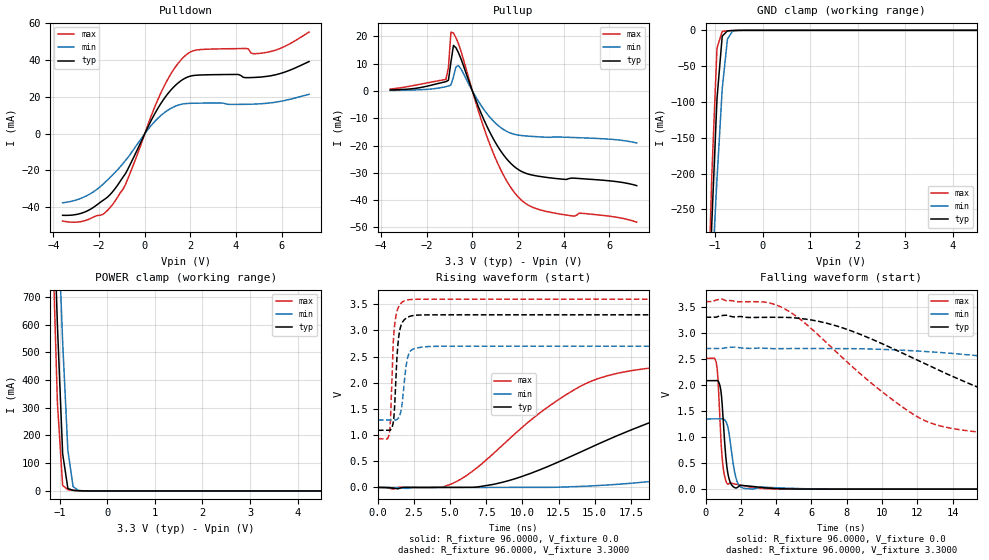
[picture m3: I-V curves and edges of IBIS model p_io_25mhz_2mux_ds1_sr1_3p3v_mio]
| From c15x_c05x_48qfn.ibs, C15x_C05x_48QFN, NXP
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[Model] p_io_25mhz_2mux_ds1_sr1_3p3v_mio
|   Model p_io_25mhz_2mux_ds1_sr1_3p3v_mio
| This model was characterised for following simulation conditions:
| External (pad) voltage:
|   - Typ: 3.3V,   - Min: 2.7V,   - Max: 3.6V
| Library cells for typ/min/max conditions are connected as defined below:
|  pad - External Pad
|  ipp_do_lv - Core Input
|  ipp_obe_lv - Output Buffer Enable
|  IOGC - NC
|  REFH3V3 - REFH3V3
|  REFL3V3 - REFL3V3
|  ZI - NC
|  abut_ncal_vddio[1] - vddio
|  abut_ncal_vddio[2] - vddio
|  abut_ncal_vddio[3] - vssio
|  abut_ncal_vddio[4] - vddio
|  abut_ncal_vddio[5] - vddio
|  abut_ncal_vddio[6] - vssio
|  abut_pcal_vddio[1] - vssio
|  abut_pcal_vddio[2] - vssio
|  abut_pcal_vddio[3] - vddio
|  abut_pcal_vddio[4] - vssio
|  abut_pcal_vddio[5] - vssio
|  abut_pcal_vddio[6] - vddio
|  ipp_do_1p8v - ipp_do_1p8v
|  ipp_dse_lv - vdd_lv
|  ipp_eftd_lv - NC
|  ipp_ina_mux_vddio - NC
|  ipp_ina_mux_vddio[0] - NC
|  ipp_ina_mux_vddio[1] - NC
|  ipp_ina_r0_vddio - NC
|  ipp_ina_r0a_vddio - NC
|  ipp_ina_r0b_vddio - NC
|  ipp_ina_r0c_vddio - NC
|  ipp_ina_r0d_vddio - NC
|  ipp_ina_r0e_vddio - NC
|  ipp_ina_r0f_vddio - NC
|  ipp_ina_r300_vddio - NC
|  ipp_ina_r300a_vddio - NC
|  ipp_ina_r300b_vddio - NC
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Model_type I/O
Polarity   Non-Inverting
Enable   Active-High
Vinl =   0.9900V
Vinh =   2.3100V
Vmeas =  1.6500V
Cref =   30.0000pF
Rref =   1.0000M
Vref =   3.3000V
C_comp   1.2811pF   1.2303pF   1.3501pF
|C_comp_pullup   0.5368pF   0.5680pF   0.5155pF
|C_comp_pulldown   0.6706pF   0.7073pF   0.6415pF
[Model Spec]
| variable   typ   min   max
Vinh   2.3100V   1.8900V   2.5200V
Vinl   0.9900V   0.8100V   1.0800V
[Temperature Range]   25.0000   0.1250k   -40.0000
[Voltage Range]   3.3000V   2.7000V   3.6000V
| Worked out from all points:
|   slope of the pulldown table from 0 to 0.495 V, typ, clamps not added: 40.8 ohm
|   slope of the pullup table from 0 to 0.495 V, typ, clamps not added: 47.8 ohm
|   GND clamp passes 1 mA (typ) near -0.74 V on its own axis
|   POWER clamp passes 1 mA (typ) near -0.62 V on its own axis
|   rising waveform, R_fixture 96.0000, V_fixture 0.0: 20-80 % time 12ns typ, 25.5ns min, 7.17ns max; typ from 0 V to 2.08 V
|   rising waveform, R_fixture 96.0000, V_fixture 3.3000: 20-80 % time 277ps typ, 348ps min, 248ps max; typ from 1.09 V to 3.3 V
|   falling waveform, R_fixture 96.0000, V_fixture 0.0: 20-80 % time 280ps typ, 355ps min, 248ps max; typ from 2.08 V to 0 V
|   falling waveform, R_fixture 96.0000, V_fixture 3.3000: 20-80 % time 9.25ns typ, 20.1ns min, 5.6ns max; typ from 3.3 V to 1.09 V
[Pulldown]
|Voltage   I(typ)   I(min)   I(max)
-3.6V     -44.37mA   -37.58mA   -47.51mA
-2.5V     -41.88mA   -33.45mA   -46.76mA
-1.84V    -36.35mA   -27.58mA   -43.92mA
-1.4V     -31.43mA   -22.29mA   -38.34mA
-850mV    -21.79mA   -14.63mA   -27.74mA
800mV     18.21mA    10.89mA    24.66mA
1.35V     26.41mA    15.03mA    36.45mA
1.9V      30.96mA    16.49mA    43.73mA
4.43V     30.52mA    16mA       46.39mA
4.76V     30.6mA     16.11mA    43.53mA
5.31V     31.15mA    16.53mA    44.19mA
7.2V      39.28mA    21.46mA    55.3mA
[Pullup]
|Voltage   I(typ)   I(min)   I(max)
-3.6V     375uA      207.1uA    721uA
-1.16V    3.419mA    1.608mA    4.218mA
-1.05V    3.929mA    1.825mA    8.684mA
-940mV    10.66mA    2.209mA    21.58mA
-830mV    16.7mA     5.227mA    21.23mA
-720mV    15.82mA    8.86mA     19.48mA
-610mV    14mA       9.299mA    17.3mA
820mV     -16.02mA   -10.13mA   -20.76mA
1.48V     -24.66mA   -14.68mA   -32.62mA
2.03V     -28.88mA   -16.19mA   -39.03mA
3.35V     -31.76mA   -16.97mA   -44.31mA
7.2V      -34.67mA   -19.04mA   -48.06mA
[GND_clamp]
|Voltage   I(typ)   I(min)   I(max)
-3.6V     -5.309A    -4.128A    -6.876A
-1.18V    -466mA     -495.4mA   -458.9mA
-1.07V    -271.1mA   -348.5mA   -204.6mA
-960mV    -95.65mA   -208mA     -24.74mA
-850mV    -8.096mA   -81.85mA   -1.471mA
-740mV    -719.7uA   -12.14mA   -717.6uA
-630mV    -272.5uA   -923.5uA   -300.8uA
-300mV    -385.6nA   -2.502uA   -74.88nA
7.2V      0A         0A         0A
[POWER_clamp]
|Voltage   I(typ)   I(min)   I(max)
-3.6V     14.48A     12.95A     16.35A
-1.16V    1.177A     1.535A     951.2mA
-1.05V    598.4mA    1.032A     318mA
-940mV    134.2mA    537.3mA    20.02mA
-830mV    8.708mA    145.4mA    4.242mA
-720mV    2.127mA    15.38mA    2.218mA
-610mV    847.4uA    1.853mA    834.1uA
7.2V      0A         0A         0A
[Ramp]
| variable   typ   min   max
dV/dt_r  1.2491/12.0373n   0.8026/25.5375n   1.5061/7.1717n
dV/dt_f  1.3249/9.2469n   0.8437/20.0855n   1.6024/5.6005n
R_load = 96.0000
[Rising Waveform]
R_fixture= 96.0000
V_fixture= 0.0
V_fixture_min= 0.0
V_fixture_max= 0.0
|time   V(typ)   V(min)   V(max)
0s        3.081nV    103.2nV    10.53nV
4.572ns   -81.02uV   -467uV     15.01mV
8.528ns   91.84mV    7.678uV    783.2mV
11.66ns   388.3mV    693.5uV    1.518V
14.79ns   773.2mV    29.16mV    2.034V
21.68ns   1.514V     196.4mV    2.356V
30.99ns   1.882V     534.2mV    2.456V
42.83ns   2.003V     937.6mV    2.493V
53.59ns   2.045V     1.127V     2.504V
127.4ns   2.082V     1.338V     2.51V
[Rising Waveform]
R_fixture= 96.0000
V_fixture= 3.3000
V_fixture_min= 2.7000
V_fixture_max= 3.6000
|time   V(typ)   V(min)   V(max)
0s        1.092V     1.289V     929.3mV
803.7ps   1.091V     1.289V     1.056V
872.4ps   1.1V       1.289V     1.314V
1.015ns   1.184V     1.289V     2.498V
1.097ns   1.316V     1.289V     2.918V
1.292ns   2.356V     1.295V     3.338V
1.568ns   3.069V     1.427V     3.511V
1.994ns   3.242V     2.393V     3.581V
2.277ns   3.276V     2.615V     3.592V
127.4ns   3.3V       2.7V       3.6V
[Falling Waveform]
R_fixture= 96.0000
V_fixture= 0.0
V_fixture_min= 0.0
V_fixture_max= 0.0
|time   V(typ)   V(min)   V(max)
0s        2.082V     1.348V     2.51V
628.2ps   2.085V     1.348V     2.384V
708.8ps   2.074V     1.348V     2.079V
818ps     1.982V     1.349V     1.278V
939ps     1.639V     1.351V     605.9mV
1.186ns   491mV      1.275V     128.8mV
1.432ns   107.4mV    825.9mV    118.9mV
1.862ns   47.89mV    93.5mV     85.59mV
3.337ns   26.85mV    36.7mV     11.08mV
127.4ns   207.6nV    4.315uV    21.7nV
[Falling Waveform]
R_fixture= 96.0000
V_fixture= 3.3000
V_fixture_min= 2.7000
V_fixture_max= 3.6000
|time   V(typ)   V(min)   V(max)
0s        3.3V       2.7V       3.6V
4.021ns   3.299V     2.697V     3.533V
7.321ns   3.144V     2.699V     2.663V
12.47ns   2.401V     2.643V     1.309V
17.53ns   1.677V     2.485V     1.041V
20.23ns   1.426V     2.369V     999.6mV
25.11ns   1.263V     2.136V     963.4mV
35.51ns   1.154V     1.674V     938.8mV
45.7ns    1.119V     1.476V     932.6mV
127.4ns   1.092V     1.294V     929.3mV
